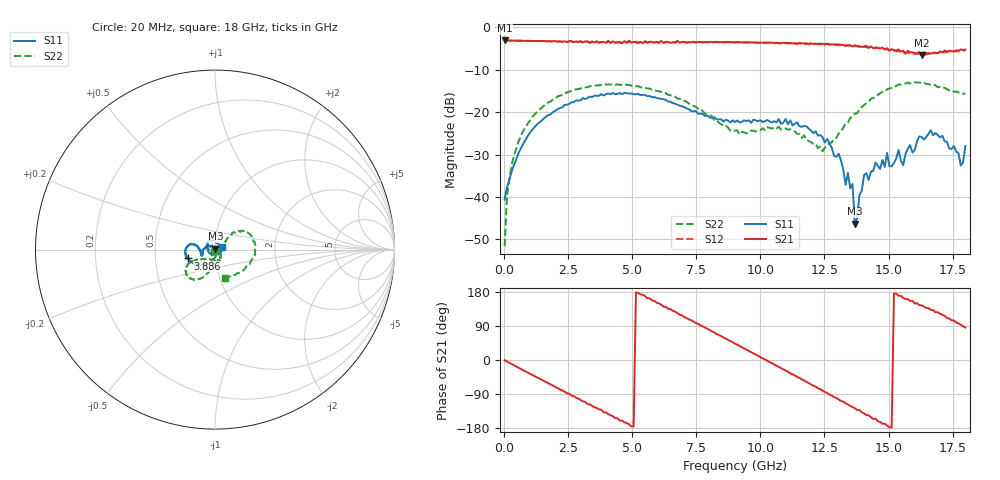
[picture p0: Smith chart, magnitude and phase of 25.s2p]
!Agilent Technologies,N5230A,US43500223,A.07.50.48
!Agilent N5230A: A.07.50.48
!Date: Monday, January 11, 2016 16:42:23
!Correction: S11(Full 2 Port(1,2))
!S21(Full 2 Port(1,2))
!S12(Full 2 Port(1,2))
!S22(Full 2 Port(1,2))
!S2P File: Measurements: S11, S21, S12, S22:
# Hz S  dB  R 50
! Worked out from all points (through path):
!   201 points, 20 MHz to 18 GHz, reference 50 ohm
!   highest |S21| = -3.08 dB at 20 MHz (marker M1); lowest = -6.5 dB at 16.29 GHz (marker M2)
!   group delay of S21, straight-line fit = 98.6 ps
!   lowest |S11| = -46.3 dB at 13.68 GHz (marker M3), VSWR 1.01, Z = 50.2 + j0.448 ohm
!   |S11| at or under -10 dB: start of sweep to end of sweep
!   |S22| runs from -51.6 to -12.9 dB; largest |S21 - S12| = 0.072
!   S11 on the Smith chart (normalised r, x): 20 MHz: 1.02, -0.00; 3.886 GHz: 0.74, -0.07; 18 GHz: 1.08, +0.03
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2e7  -40.61 -4.2  -3.08 -0.7  -3.08 -0.9  -51.58 -22.4
1.099e8  -37.68 -29.2  -3.09 -4.0  -3.10 -4.2  -40.19 -54.3
2.897e8  -34.10 -55.9  -3.11 -10.5  -3.13 -10.7  -32.51 -75.3
7.392e8  -27.54 -88.9  -3.15 -26.7  -3.15 -26.8  -24.51 -89.9
3.0766e9  -16.68 -148.2  -3.56 -109.4  -3.47 -109.8  -14.15 -120.7
3.8857e9  -16.05 -161.8  -3.42 -138.1  -3.51 -138.5  -13.62 -130.3
6.0433e9  -16.76 169.2  -3.58 149.6  -3.72 147.2  -15.06 -151.0
7.5716e9  -20.39 170.2  -3.44 95.5  -3.41 93.2  -19.17 -149.1
9.01e9  -22.32 -163.9  -3.54 43.4  -3.55 40.4  -24.35 -113.7
1.04484e10  -22.41 -159.6  -3.60 -8.3  -3.66 -12.1  -23.89 -69.1
1.20666e10  -24.92 175.5  -3.91 -67.5  -3.81 -71.1  -27.42 -37.3
1.30555e10  -29.78 141.0  -4.01 -104.0  -4.22 -108.5  -25.02 30.6
1.33252e10  -37.13 141.5  -4.24 -114.6  -4.44 -118.5  -22.60 36.2
1.34151e10  -34.29 126.5  -4.22 -117.1  -4.23 -121.4  -22.44 39.5
1.35949e10  -36.91 65.6  -4.50 -123.6  -4.54 -128.6  -20.98 42.3
1.36848e10  -46.30 67.3  -4.21 -127.5  -4.47 -130.6  -20.35 42.8
1.40444e10  -34.89 -3.1  -4.58 -141.0  -4.50 -145.3  -18.32 43.3
1.50333e10  -32.73 -79.0  -5.49 -178.0  -5.45 178.5  -14.43 33.1
1.62919e10  -25.85 147.2  -6.54 144.1  -6.26 138.7  -13.05 -2.6
1.7101e10  -25.56 102.7  -5.87 119.4  -5.94 114.2  -14.23 -36.4
1.78202e10  -32.57 35.9  -5.17 93.0  -5.68 87.0  -15.47 -64.3
1.8e10  -27.96 17.5  -5.21 85.9  -5.52 79.5  -15.61 -70.6
